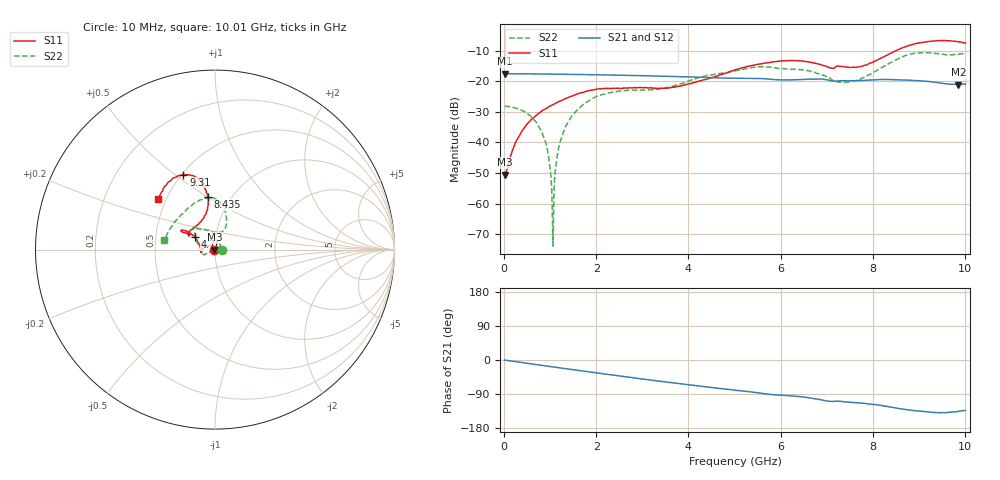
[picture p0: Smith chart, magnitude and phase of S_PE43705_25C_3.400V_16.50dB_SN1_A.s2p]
! Device ID: PE43705
! Serial: 1
! Insertion: A
! Impedance: 50 ohm
! Temp: 25C
! VDD: 3.400V
! Attenuation Step: 16.50dB
#  Hz  S  RI  R  50
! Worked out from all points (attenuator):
!   401 points, 10 MHz to 10.01 GHz, reference 50 ohm
!   highest |S21| = -17.54 dB at 10 MHz (marker M1); lowest = -21.1 dB at 9.86 GHz (marker M2)
!   lowest |S11| = -50.5 dB at 10 MHz (marker M3), VSWR 1.01, Z = 49.7 + j0.0339 ohm
!   |S11| at or under -10 dB: start of sweep to 8.512 GHz
!   |S22| runs from -73.8 to -10.7 dB; largest |S21 - S12| = 0.0015
!   S11 on the Smith chart (normalised r, x): 10 MHz: 0.99, +0.00; 4.76 GHz: 0.79, +0.11; 8.435 GHz: 0.78, +0.50; 9.31 GHz: 0.51, +0.54; 10.01 GHz: 0.45, +0.31
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1e7  -0.00298 0.000341  0.1327 -0.000561  0.1328 -0.000521  0.039 4.88e-05
3.35e8  -0.00562 0.0117  0.131 -0.0136  0.1309 -0.0135  0.0344 0.004
7.6e8  -0.0213 0.0213  0.1276 -0.0299  0.1276 -0.0297  0.017 0.00502
9.35e8  -0.0295 0.0217  0.1254 -0.0364  0.1255 -0.0363  0.00739 0.00259
9.85e8  -0.0324 0.0216  0.1248 -0.0382  0.1248 -0.0382  0.00428 0.00142
1.01e9  -0.0334 0.0212  0.1244 -0.0391  0.1243 -0.039  0.00302 0.000788
1.06e9  -0.0359 0.021  0.1235 -0.0409  0.1236 -0.0408  -0.000183 8.82e-05
1.11e9  -0.0383 0.02  0.1229 -0.0425  0.1228 -0.0424  -0.00324 -0.00142
1.16e9  -0.0408 0.0197  0.1222 -0.0442  0.1221 -0.0441  -0.00608 -0.00226
1.26e9  -0.0453 0.018  0.1205 -0.0477  0.1206 -0.0476  -0.012 -0.00468
1.685e9  -0.0644 0.00757  0.1126 -0.0615  0.1126 -0.0615  -0.0365 -0.0162
2.285e9  -0.0752 -0.0109  0.0986 -0.0784  0.0988 -0.0784  -0.0578 -0.0287
3.36e9  -0.0759 -0.00728  0.068 -0.0999  0.0682 -0.0998  -0.074 -0.00487
4.76e9  -0.1115 0.0694  0.0266 -0.1094  0.0269 -0.1094  -0.11 0.0815
5.01e9  -0.1276 0.0844  0.02 -0.1096  0.0203 -0.1097  -0.1142 0.0941
6.685e9  -0.1764 0.0952  -0.0208 -0.1059  -0.0209 -0.1059  -0.084 0.1145
7.435e9  -0.1221 0.1182  -0.0364 -0.0952  -0.0362 -0.0953  0.0124 0.0962
8.36e9  -0.0369 0.2765  -0.059 -0.0886  -0.0591 -0.0892  0.0626 0.186
8.435e9  -0.0393 0.2939  -0.0611 -0.0867  -0.0614 -0.0873  0.0603 0.2008
9.31e9  -0.1764 0.4174  -0.0721 -0.0643  -0.0719 -0.0642  -0.0916 0.2718
9.86e9  -0.2911 0.326  -0.0631 -0.0616  -0.063 -0.0612  -0.2457 0.1218
1.001e10  -0.3153 0.2797  -0.0613 -0.0658  -0.0626 -0.0661  -0.2843 0.0543
